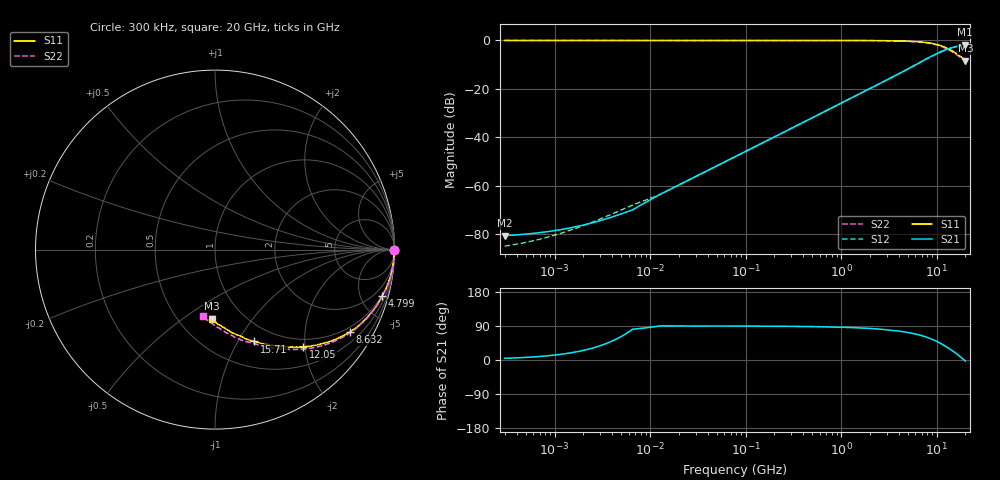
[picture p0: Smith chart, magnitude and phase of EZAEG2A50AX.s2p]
!*** S-Parameter ***
!Copyright (C)  Panasonic Industry
!ESD Suppressor
!Parts No.  EZAEG2A50AX
! Size : 1005mm
# hz S ma R 50
! 2 Port Network Data from SP1.SP block
! freq  magS11  angS11  magS21  angS21  magS12  angS12  magS22  angS22
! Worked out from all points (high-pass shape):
!   966 points, 300 kHz to 20 GHz, reference 50 ohm
!   highest |S21| = -1.80 dB at 19.77 GHz (marker M1); lowest = -80.7 dB at 300 kHz (marker M2)
!   |S21| within 3 dB of the highest: 10.87 GHz to end of sweep
!   lowest |S11| = -8.3 dB at 20 GHz (marker M3), VSWR 2.25, Z = 36 - j32.5 ohm
!   |S11| at or under -10 dB: nowhere
!   |S22| runs from -8.5 to 0.0 dB; largest |S21 - S12| = 0.022
!   S11 on the Smith chart (normalised r, x): 300 kHz: open; 4.799 GHz: 0.91, -7.18; 8.632 GHz: 0.82, -3.35; 12.05 GHz: 0.84, -1.96; 15.71 GHz: 0.79, -1.17; 20 GHz: 0.72, -0.65
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300000  1 -0.0  9.21e-05 4.4  5.589e-05 -158.1  1 -0.0
533414.4  1 -0.0  0.0001004 7.3  6.868e-05 -162.3  1 -0.0
1088917  1 -0.0  0.0001202 14.1  9.914e-05 -172.4  1 -0.0
1913988  1 -0.0  0.0001496 24.3  0.0001444 172.7  1 -0.0
3442560  1 -0.0  0.0002041 43.0  0.0002282 145.1  1 -0.0
6263581  1 -0.0  0.0003046 77.7  0.0003829 94.1  0.9999 -0.0
1.221117e7  1 -0.0  0.0006296 89.4  0.0006369 89.4  1 -0.0
7.790674e7  0.9987 -0.2  0.003962 89.5  0.003955 89.5  1 -0.2
4.970419e8  0.9986 -1.5  0.02511 88.2  0.0251 88.1  0.9997 -1.5
1.483493e9  0.9958 -4.5  0.07482 85.0  0.07478 84.8  0.997 -4.8
2.271139e9  0.9919 -7.0  0.1148 82.3  0.1147 82.2  0.9927 -7.5
3.171107e9  0.9858 -10.0  0.1611 79.3  0.1606 79.0  0.9851 -10.6
4.799215e9  0.9665 -15.6  0.2466 73.3  0.2459 72.9  0.965 -16.6
6.624278e9  0.9342 -22.8  0.348 65.7  0.3453 65.6  0.93 -24.2
8.632022e9  0.8796 -31.6  0.4629 56.0  0.4561 56.3  0.8701 -33.7
1.049768e10  0.8029 -40.3  0.5578 46.3  0.5499 46.5  0.7893 -43.3
1.205257e10  0.7302 -47.9  0.6271 37.8  0.6149 38.1  0.7103 -51.6
1.399797e10  0.6361 -57.8  0.6939 27.6  0.6845 28.4  0.6119 -62.5
1.570557e10  0.5563 -66.8  0.7446 19.1  0.7312 19.3  0.5332 -72.4
1.762148e10  0.4745 -78.2  0.7877 8.6  0.7718 9.4  0.4512 -84.5
1.977111e10  0.3948 -91.3  0.8131 -2.2  0.7966 -1.2  0.3815 -99.4
2e10  0.3852 -92.6  0.812 -3.0  0.798 -2.3  0.3778 -100.1
